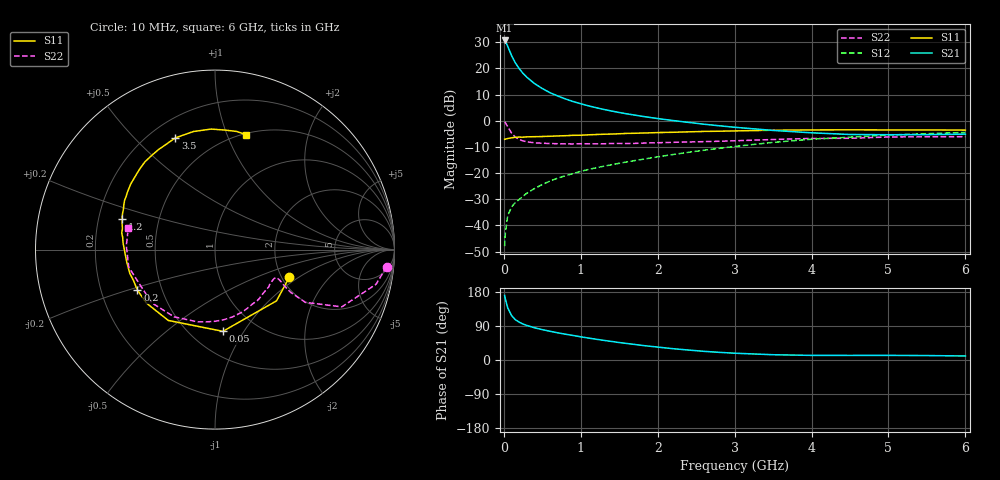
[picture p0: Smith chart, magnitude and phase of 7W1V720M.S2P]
! Infineon Technologies  Discrete & RF Semiconductors
! BFS17W
! Si NPN RF Bipolar Junction Transistor in SOT323
! VCE = 1.75 V  IC = 20 mA
! Common Emitter S-Parameters:  August  1999
# GHz  S  MA  R  50
!  f  S11  S21  S12  S22
! GHz  MAG  ANG  MAG  ANG  MAG  ANG  MAG  ANG
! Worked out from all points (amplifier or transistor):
!   36 points, 10 MHz to 6 GHz, reference 50 ohm
!   highest |S21| = 30.7 dB at 10 MHz (marker M1)
!   |S21| within 3 dB of that: start of sweep to 61.21 MHz
!   unconditionally stable (mu >= 1): 227 MHz to 3.162 GHz; 3.704 GHz to end of sweep
!   at 250 MHz: K = 1.05, MAG = 22.2 dB, |S12| = -28.8 dB
!   at 1.4 GHz: K = 1.25, MAG = 7.3 dB, |S12| = -16.8 dB
!   at 6 GHz: K = 1.10, MAG = -2.2 dB, |S12| = -4.5 dB
!   S11 on the Smith chart (normalised r, x): 10 MHz: 2.19, -0.84; 50 MHz: 0.70, -0.81; 200 MHz: 0.36, -0.22; 1.2 GHz: 0.30, +0.15; 3.5 GHz: 0.30, +0.66; 6 GHz: 0.51, +1.17
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0.01  0.442 -20.5  34.38 170.5  0.004 79.9  0.9606 -5.7
0.02  0.4461 -39.8  33.13 160.6  0.0072 75.5  0.9184 -12.1
0.05  0.4575 -84.5  26.67 137.9  0.0153 62.7  0.7753 -24.3
0.1  0.4727 -123.4  17.74 117.3  0.0224 56.3  0.5826 -30.3
0.15  0.4846 -142.1  12.8 106.4  0.0274 55.9  0.4862 -29.5
0.2  0.4877 -152.3  9.932 99.8  0.0313 59.2  0.4398 -27.8
0.25  0.4859 -159.4  8.064 94.9  0.0361 59.6  0.4116 -26.1
0.3  0.4928 -164.4  6.78 91.1  0.0413 62.5  0.397 -25.2
0.4  0.4965 -171.8  5.142 85.0  0.0508 65.0  0.3787 -24.5
0.5  0.5005 -176.7  4.135 80.1  0.0603 66.3  0.3721 -24.8
0.6  0.506 179.4  3.448 75.8  0.0704 67.1  0.3673 -25.9
0.7  0.5133 176.0  2.981 71.8  0.0801 67.7  0.364 -27.8
0.9  0.5276 169.9  2.335 64.7  0.0978 68.5  0.3611 -32.5
1.1  0.5392 163.9  1.931 57.9  0.1172 68.6  0.3629 -38.0
1.2  0.546 161.7  1.78 54.8  0.1262 68.5  0.3623 -41.0
1.6  0.5736 151.4  1.357 43.5  0.1633 68.1  0.3677 -54.1
2.2  0.6031 137.6  1.011 29.8  0.2265 66.7  0.3874 -75.3
2.8  0.6318 124.1  0.803 20.2  0.2971 62.7  0.4057 -96.9
3.5  0.6604 109.5  0.654 13.9  0.3864 55.5  0.4386 -121.4
4.5  0.6718 91.9  0.547 12.1  0.4864 42.2  0.4623 -155.3
5.5  0.6692 79.5  0.543 11.7  0.5664 30.2  0.4945 177.6
6  0.663 74.7  0.556 10.6  0.5985 24.4  0.4982 165.7
